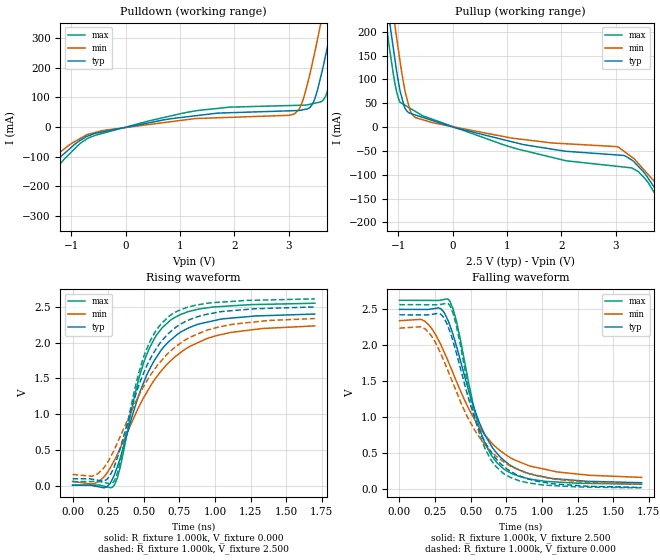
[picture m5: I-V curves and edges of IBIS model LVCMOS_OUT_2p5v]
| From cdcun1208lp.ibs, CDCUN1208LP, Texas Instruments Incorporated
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[Model]   LVCMOS_OUT_2p5v
Model_type   Output
Polarity   Non-Inverting
Enable   Active-High
Vmeas = 1.25
Vref = 1.25
Cref = 0pF
Rref = 50
|   typ   min   max
C_comp   6.1385pF   5.8664pF   6.2817pF
[Voltage Range]   2.5   2.375   2.625
[Temperature Range]   27   105   -40
[Pullup Reference]   2.5   2.375   2.625
[Pulldown Reference]   -0   -0   0
[Power Clamp Reference]   2.5   2.375   2.625
[GND Clamp Reference]   0   0   0
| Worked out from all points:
|   slope of the pulldown table from 0 to 0.375 V, typ, clamps not added: 27.7 ohm
|   slope of the pullup table from 0 to 0.375 V, typ, clamps not added: 34.9 ohm
|   falling waveform, R_fixture 1.000k, V_fixture 2.500: 20-80 % time 259ps typ, 356ps min, 191ps max; typ from 2.49 V to 0.082 V
|   rising waveform, R_fixture 1.000k, V_fixture 0.000: 20-80 % time 283ps typ, 390ps min, 209ps max; typ from 0.005 V to 2.4 V
|   rising waveform, R_fixture 1.000k, V_fixture 2.500: 20-80 % time 280ps typ, 386ps min, 207ps max; typ from 0.095 V to 2.5 V
|   falling waveform, R_fixture 1.000k, V_fixture 0.000: 20-80 % time 255ps typ, 348ps min, 188ps max; typ from 2.42 V to 0.016 V
[Pulldown]
|   Voltage   I(typ)   I(min)   I(max)
-2.5V     -776.1mA   -667.9mA   -877.9mA
-2.123V   -427.8mA   -331.9mA   -520.7mA
-1.928V   -270.1mA   -203.8mA   -346.5mA
-1.736V   -201.1mA   -160.8mA   -241.9mA
-710.5mV  -31.18mA   -25.36mA   -39.5mA
1.317V    38.9mA     28.98mA    55.7mA
3.106V    55.38mA    44.65mA    73.04mA
3.388V    66.08mA    178.7mA    76.92mA
3.578V    162.3mA    340.6mA    84.39mA
3.795V    346.3mA    539.6mA    180.3mA
3.98V     518.4mA    714.9mA    341mA
4.992V    1.498A     1.694A     1.318A
[Pullup]
|   Voltage   I(typ)   I(min)   I(max)
-2.5V     1.505A     1.579A     1.448A
-1.212V   268.7mA    345.5mA    209.8mA
-1.134V   200.9mA    276.3mA    145.6mA
-1.058V   140.4mA    211.4mA    90.23mA
-885.3mV  42.06mA    82.19mA    46.56mA
-682.9mV  25.27mA    19.97mA    32.77mA
1.186V    -33.53mA   -24.5mA    -45.84mA
3.024V    -58.52mA   -41.07mA   -82.33mA
3.418V    -82.62mA   -76.51mA   -93.62mA
4.222V    -213.7mA   -187.9mA   -240.3mA
4.301V    -229.7mA   -209.4mA   -257.6mA
4.992V    -769.9mA   -778.9mA   -751.7mA
[Ramp]
R_load = 1000
|   typ   min   max
dV/dt_r   1.436/2.83354e-010   1.33919/3.89579e-010   1.52747/2.08383e-010
dV/dt_f   1.447/2.58584e-010   1.35279/3.55319e-010   1.53483/1.90062e-010
[Falling Waveform]
R_fixture = 1.000k
V_fixture = 2.500
V_fixture_min = 2.375
V_fixture_max = 2.625
C_fixture = 0.000
|  time   V(typ)   V(min)   V(max)
0s        2.494V     2.336V     2.62V
180.2ps   2.493V     2.327V     2.619V
290.3ps   2.503V     2.003V     2.623V
353.9ps   2.272V     1.715V     2.608V
401.4ps   1.975V     1.487V     2.32V
511ps     1.2V       1.021V     1.232V
568.4ps   883.7mV    831.3mV    802.6mV
732.2ps   396.1mV    492.2mV    273.3mV
1.058ns   145.8mV    252.9mV    96.9mV
1.7ns     82.04mV    155.9mV    61.53mV
[Rising Waveform]
R_fixture = 1.000k
V_fixture = 0.000
V_fixture_min = 0.000
V_fixture_max = 0.000
C_fixture = 0.000
|  time   V(typ)   V(min)   V(max)
0s        5.309mV    59.3mV     4.486mV
185.2ps   -18.47mV   55.49mV    6.579mV
242.2ps   -14.14mV   176.8mV    -17.93mV
295ps     158.4mV    358.3mV    13.12mV
333.7ps   380.1mV    519.8mV    249.6mV
497.9ps   1.434V     1.226V     1.712V
580ps     1.769V     1.493V     2.075V
685.6ps   2.03V      1.74V      2.31V
1.007ns   2.313V     2.095V     2.5V
1.7ns     2.399V     2.233V     2.55V
[Rising Waveform]
R_fixture = 1.000k
V_fixture = 2.500
V_fixture_min = 2.375
V_fixture_max = 2.625
C_fixture = 0.000
|  time   V(typ)   V(min)   V(max)
0s        94.77mV    155.9mV    55.22mV
175.1ps   75.86mV    161.8mV    57.31mV
237.2ps   80.05mV    300mV      35.58mV
293ps     266.5mV    501.4mV    67.42mV
331.3ps   495.8mV    672.7mV    304.2mV
492.4ps   1.542V     1.364V     1.76V
578.4ps   1.886V     1.634V     2.145V
675.8ps   2.132V     1.859V     2.365V
1.026ns   2.426V     2.217V     2.564V
1.7ns     2.498V     2.336V     2.611V
[Falling Waveform]
R_fixture = 1.000k
V_fixture = 0.000
V_fixture_min = 0.000
V_fixture_max = 0.000
C_fixture = 0.000
|  time   V(typ)   V(min)   V(max)
0s        2.418V     2.233V     2.559V
180.2ps   2.417V     2.223V     2.558V
290.3ps   2.426V     1.876V     2.563V
353.9ps   2.186V     1.574V     2.547V
397.5ps   1.903V     1.361V     2.283V
560.1ps   819.2mV    718.7mV    772.1mV
636.2ps   531.1mV    530.8mV    420.5mV
723.2ps   325mV      384.3mV    221.6mV
1.058ns   72.22mV    141mV      44.08mV
1.7ns     15.84mV    59.3mV     10.56mV
